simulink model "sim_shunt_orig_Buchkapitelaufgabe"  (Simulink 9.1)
settings: Solver=ode23s  StartTime=0.0  StopTime=4000  RelTol=1e-8  EnableMultiTasking=on
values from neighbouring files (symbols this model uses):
  Bauchdruck = 0    [InitVentil_Buchkapitel.m]
  HydrHoehe = sin(Liegewinkel)*l_Schlauch*73.55    [InitVentil_Buchkapitel.m]
  ICP_n = 0.9330    (= 0.933)    [InitVentil_Buchkapitel.m]
  ICP_shift = 9*sin(Liegewinkel*2 + pi/2)+5 - 14    [InitVentil_Buchkapitel.m]
  R_hyd = 128*eta_Liquor*l_Schlauch/(pi*d_Schlauch^4)*Umrechnungsfaktor    (= 68180382716.6)    [InitVentil_Buchkapitel.m]
  ventil_oeffn = 7    [InitVentil_Buchkapitel.m]
undefined symbols (not defined in the file or in its folder): ABP_n, alph, alphco2, G_vor, h_01, h_02, h_0_ven, ini1_reg, ini2_reg, K_e1, K_e2, K_e_ven, K_G1, K_G2, K_G_ven, k_prod, k_res, K_v1, K_v2, K_v_ven, n_m1, n_m2, O2_verb, p1_n, Pco2_AB, PCO2_soll, Po2_ab, PO2_blut, PO2_soll, r1_100, r2_100, r2_n, r_01, r_02, r_0_ven, r_m1, r_m2, r_t1, r_t2, rv_100, sigma_01, sigma_02, sigma_0_ven, sigma_0_visk_1, sigma_0_visk_2, sigma_koll1, sigma_koll2, sigma_koll_ven, sigma_m01, sigma_m02, V, V1_n, V2_n, V_ven_0, VBPss_n
libraries: neural x36, simulink_extras x3, simulink x1
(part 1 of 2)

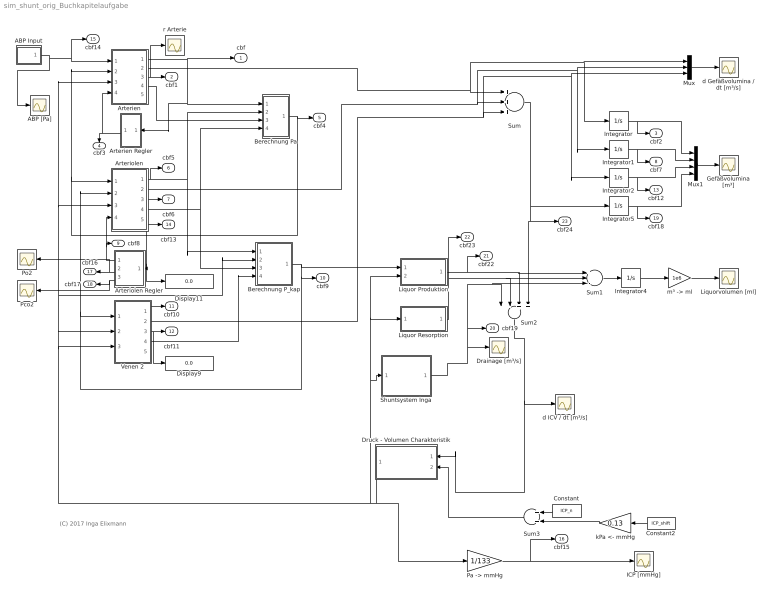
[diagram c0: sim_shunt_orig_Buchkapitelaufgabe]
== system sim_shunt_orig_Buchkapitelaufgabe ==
  note: (C) 2017 Inga Elixmann
  ABP Input : Subsystem
  ABP [Pa] : Scope
  Arterien : Subsystem
  Arterien Regler : Subsystem
  Arteriolen : Subsystem
  Arteriolen Regler : Subsystem
  Berechnung P_kap : Subsystem
  Berechnung Pa : Subsystem
  Constant : Constant  Value=ICP_n
  Constant2 : Constant  Value=ICP_shift
  Display11 : Display
  Display9 : Display
  Drainage [m³/s] : Scope
  Druck - Volumen Charakteristik : Subsystem
  Gefäßvolumina [m³] : Scope
  ICP [mmHg] : Scope
  Integrator : Integrator  InitialCondition=V1_n*1e-6
  Integrator1 : Integrator  InitialCondition=V2_n*1e-6
  Integrator2 : Integrator  InitialCondition=V_ven_0*1e-6
  Integrator4 : Integrator  InitialCondition=150*1e-6
  Integrator5 : Integrator  InitialCondition=(V_ven_0+V2_n+V1_n)*1e-6
  Liquor Produktion : Subsystem
  Liquor Resorption : Subsystem
  Liquorvolumen [ml] : Scope
  Mux : Mux  Inputs=3
  Mux1 : Mux
  "Pa -> mmHg" : Gain  Gain=1/133
  Pco2 : Scope
  Po2 : Scope
  Shuntsystem Inga : Subsystem
  Sum : Sum  Inputs=+++
  Sum1 : Sum  Inputs=+--
  Sum2 : Sum  Inputs=--++
  Sum3 : Sum
  Venen 2 : Subsystem
  d Gefäßvolumina / dt [m³/s] : Scope
  d ICV / dt [m³/s] : Scope
  kPa <- mmHg : Gain  Gain=0.13
  "m³ -> ml" : Gain  Gain=1e6
  r Arterie : Scope
  cbf : Outport
  cbf1 : Outport  Port=2
  cbf2 : Outport  Port=3
  cbf3 : Outport  Port=4
  cbf4 : Outport  Port=5
  cbf5 : Outport  Port=6
  cbf6 : Outport  Port=7
  cbf7 : Outport  Port=8
  cbf8 : Outport  Port=9
  cbf9 : Outport  Port=10
  cbf10 : Outport  Port=11
  cbf11 : Outport  Port=12
  cbf12 : Outport  Port=13
  cbf13 : Outport  Port=14
  cbf14 : Outport  Port=15
  cbf15 : Outport  Port=16
  cbf16 : Outport  Port=17
  cbf17 : Outport  Port=18
  cbf18 : Outport  Port=19
  cbf19 : Outport  Port=20
  cbf22 : Outport  Port=21
  cbf23 : Outport  Port=22
  cbf24 : Outport  Port=23
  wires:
  Arterien/4(G1) -> Berechnung Pa/3(G1)
  Arteriolen/4(G2) -> Berechnung Pa/4(G2), Berechnung P_kap/3(G2)
  Arterien/3(r1) -> cbf1/1, r Arterie/1
  Arterien Regler/1(A1) -> Arterien/4(A), cbf3/1
  Berechnung Pa/1(Pa) -> cbf4/1, Arterien/2(P2), Arteriolen/1(P1)
  Arteriolen/1(PI2) -> Berechnung Pa/2(PI2), Berechnung P_kap/1(PI2), cbf5/1
  Arteriolen/3(r2) -> cbf6/1
  Venen 2/1(PI_ven) -> cbf10/1
  ABP Input/1(ABP) -> Arterien/1(P1), cbf14/1, ABP [Pa]/1
  Venen 2/3(r_ven) -> cbf11/1, Display9/1
  Integrator/1 -> cbf2/1, Mux1/1
  Arterien/2(dV1) -> Sum/1, Mux/1, Integrator/1
  Integrator1/1 -> cbf7/1, Mux1/2
  Arteriolen/2(dV2) -> Sum/2, Mux/2, Integrator1/1
  Integrator2/1 -> Mux1/3, cbf12/1
  Venen 2/4(G_ven) -> Berechnung P_kap/4(G_pv)
  Berechnung P_kap/1(P_kap) -> Liquor Produktion/1(P_kap), Venen 2/1(P1), Arteriolen/2(P2), cbf9/1
  Venen 2/2(dV_ven) -> Sum/3, Mux/3, Integrator2/1
  Arteriolen/5(cbf2) -> cbf13/1, Display11/1, Arteriolen Regler/1(CBF)
  Arteriolen Regler/1(A2) -> Arteriolen/4(A), cbf8/1
  Arteriolen Regler/2(Po2) -> cbf16/1, Po2/1
  Arteriolen Regler/3(Pco2) -> cbf17/1, Pco2/1
  Arterien/1(PI1) -> cbf/1, Berechnung Pa/1(PI1), Arterien Regler/1(Pa)
  Druck - Volumen Charakteristik/1(ICP) -> "Pa -> mmHg"/1, Venen 2/2(P2), Arterien/3(ICP), Arteriolen/3(ICP), Berechnung P_kap/2(ICP), Venen 2/3(ICP), Shuntsystem Inga/1(ICP), Liquor Resorption/1(ICP), Liquor Produktion/2(ICP)
  Liquor Produktion/1(dV_prod) -> Sum1/1, Sum2/3, cbf22/1
  Liquor Resorption/1(dV_res) -> Sum1/2, Sum2/2, cbf23/1
  Sum2/1 -> Druck - Volumen Charakteristik/1(dV/dt), d ICV / dt [m³/s]/1
  Sum/1 -> Integrator5/1, Sum2/4, cbf24/1
  Mux/1 -> d Gefäßvolumina / dt [m³/s]/1
  "Pa -> mmHg"/1 -> ICP [mmHg]/1, cbf15/1
  Mux1/1 -> Gefäßvolumina [m³]/1
  Sum1/1 -> Integrator4/1
  Integrator4/1 -> "m³ -> ml"/1
  "m³ -> ml"/1 -> Liquorvolumen [ml]/1
  Integrator5/1 -> cbf18/1, Mux1/4
  Constant/1 -> Sum3/1
  Sum3/1 -> Druck - Volumen Charakteristik/2(ICP_start)
  Constant2/1 -> kPa <- mmHg/1
  kPa <- mmHg/1 -> Sum3/2
  Shuntsystem Inga/1(dV_shunt) -> Drainage [m³/s]/1, Sum1/3, Sum2/1, cbf19/1

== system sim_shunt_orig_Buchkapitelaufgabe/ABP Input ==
  note: Vereinfachte Annahme: konstanter ABP
  ABP Generator : Subsystem
  ABP [kPa] : Display
  Constant : Constant  Value=ABP_n
  Constant1 : Constant
  From Workspace : FromWorkspace  VariableName=[T,U]  SampleTime=0  Interpolate=off  OutputAfterFinalValue=Holding final value
  Manual Switch : ManualSwitch  CurrentSetting=0
  Manual Switch1 : ManualSwitch
  Manual Switch2 : ManualSwitch
  Product : Product
  Slider Gain : simulink/Math Operations/Slider Gain  gain=1  low=0  high=2
  Step : Step  Time=20  Before=1  After=1.3  SampleTime=0
  "kPa -> Pa" : Gain  Gain=1000
  ABP : Outport
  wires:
  Constant/1 -> Slider Gain/1
  Manual Switch/1 -> Product/2
  Slider Gain/1 -> Product/1
  Step/1 -> Manual Switch/1
  Manual Switch1/1 -> Manual Switch/2
  From Workspace/1 -> Manual Switch1/2
  Constant1/1 -> Manual Switch1/1
  Product/1 -> Manual Switch2/1
  ABP Generator/1(ABP) -> Manual Switch2/2
  Manual Switch2/1 -> ABP [kPa]/1, "kPa -> Pa"/1
  "kPa -> Pa"/1 -> ABP/1

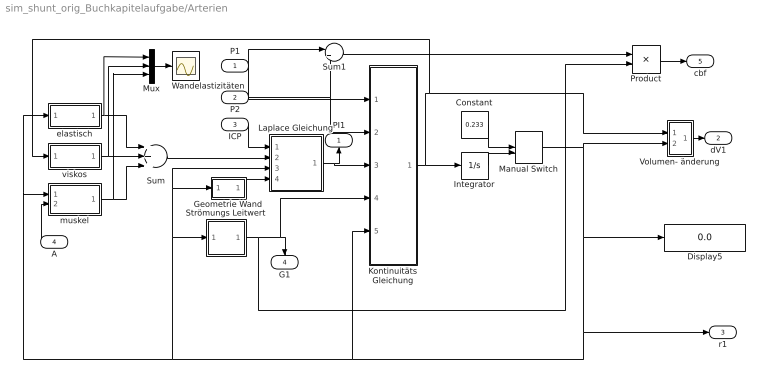
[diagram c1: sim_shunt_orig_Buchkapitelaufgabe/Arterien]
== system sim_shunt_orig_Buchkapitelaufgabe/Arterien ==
  P1 : Inport
  P2 : Inport  Port=2
  ICP : Inport  Port=3
  A : Inport  Port=4
  Constant : Constant  Value=0.233
  Display5 : Display
  Geometrie Wand : Subsystem
  Integrator : Integrator  InitialCondition=r1_100*0.01
  Kontinuitäts Gleichung : Subsystem
  Laplace Gleichung : Subsystem
  Manual Switch : ManualSwitch  CurrentSetting=0
  Mux : Mux  Inputs=3
  Product : Product
  Strömungs Leitwert : Subsystem
  Sum : Sum  Inputs=+++
  Sum1 : Sum  Inputs=|+-
  Volumen- änderung : Subsystem
  Wandelastizitäten : Scope
  elastisch : Subsystem
  muskel : Subsystem
  viskos : Subsystem
  PI1 : Outport
  dV1 : Outport  Port=2
  r1 : Outport  Port=3
  G1 : Outport  Port=4
  cbf : Outport  Port=5
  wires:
  ICP/1 -> Laplace Gleichung/1(ICP)
  Laplace Gleichung/1(PI) -> Kontinuitäts Gleichung/3(PI), PI1/1
  Geometrie Wand/1(h) -> Laplace Gleichung/4(h)
  Constant/1 -> Manual Switch/1
  Integrator/1 -> Manual Switch/2
  Volumen- änderung/1(dV) -> dV1/1
  Manual Switch/1 -> Volumen- änderung/2(r), Strömungs Leitwert/1(r), Geometrie Wand/1(r), Laplace Gleichung/3(r), muskel/1(r), elastisch/1(r), Kontinuitäts Gleichung/5(r), r1/1, Display5/1
  Kontinuitäts Gleichung/1(dr) -> Integrator/1, Volumen- änderung/1(dr), viskos/1(dr)
  A/1 -> muskel/2(A)
  Sum/1 -> Laplace Gleichung/2(Sigma)
  Product/1 -> cbf/1
  P1/1 -> Kontinuitäts Gleichung/1(P1), Sum1/1
  P2/1 -> Kontinuitäts Gleichung/2(P2), Sum1/2
  Sum1/1 -> Product/1
  Strömungs Leitwert/1(G) -> G1/1, Kontinuitäts Gleichung/4(G), Product/2
  elastisch/1(sigma_e) -> Sum/1, Mux/1
  viskos/1(sigma_v) -> Sum/2, Mux/2
  muskel/1(sigma_m) -> Sum/3, Mux/3
  Mux/1 -> Wandelastizitäten/1

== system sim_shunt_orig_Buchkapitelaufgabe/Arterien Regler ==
  Pa : Inport
  CBF Norm : Constant  Value=p1_n
  Display4 : Display
  Gain : Gain  Gain=10
  Gain1 : Gain  Gain=0
  Gain2 : Gain  Gain=1/p1_n
  Integrator1 : Integrator  InitialCondition=ini1_reg  LimitOutput=on  UpperSaturationLimit=100  LowerSaturationLimit=-100
  Mux : Mux  Inputs=3
  "Pa -> kPa" : Gain  Gain=0.001
  Scope : Scope
  Sum1 : Sum  Inputs=|+-
  Sum2 : Sum  Inputs=|++
  Transfer Fcn (with initial outputs) : simulink_extras/Additional Linear/Transfer Fcn (with initial outputs)  N=[1]  D=[2 1]  Y0=A1_100  U0=A1_100
  Transfer Fcn (with initial outputs)1 : simulink_extras/Additional Linear/Transfer Fcn (with initial outputs)  N=[1]  D=[2 1]  Y0=A1_100  U0=A1_100
  logsig2 : neural/Transfer Functions/logsig
  A1 : Outport
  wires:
  Gain/1 -> Sum2/2
  logsig2/1 -> Transfer Fcn (with initial outputs)/1
  Gain1/1 -> Integrator1/1
  Integrator1/1 -> Sum2/1
  Sum2/1 -> logsig2/1, Display4/1
  Transfer Fcn (with initial outputs)1/1 -> A1/1
  Transfer Fcn (with initial outputs)/1 -> Transfer Fcn (with initial outputs)1/1
  Pa/1 -> "Pa -> kPa"/1
  CBF Norm/1 -> Sum1/2, Mux/2
  Sum1/1 -> Gain2/1
  Gain2/1 -> Gain/1, Gain1/1, Mux/3
  Mux/1 -> Scope/1
  "Pa -> kPa"/1 -> Sum1/1, Mux/1

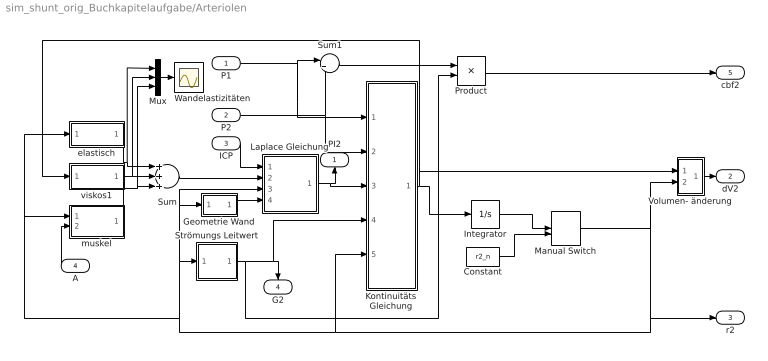
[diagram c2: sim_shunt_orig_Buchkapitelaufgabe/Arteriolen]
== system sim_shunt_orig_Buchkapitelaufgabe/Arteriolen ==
  P1 : Inport
  P2 : Inport  Port=2
  ICP : Inport  Port=3
  A : Inport  Port=4
  Constant : Constant  Value=r2_n
  Geometrie Wand : Subsystem
  Integrator : Integrator  InitialCondition=r2_100*0.01
  Kontinuitäts Gleichung : Subsystem
  Laplace Gleichung : Subsystem
  Manual Switch : ManualSwitch
  Mux : Mux  Inputs=3
  Product : Product
  Strömungs Leitwert : Subsystem
  Sum : Sum  Inputs=+++
  Sum1 : Sum  Inputs=|+-
  Volumen- änderung : Subsystem
  Wandelastizitäten : Scope
  elastisch : Subsystem
  muskel : Subsystem
  viskos1 : Subsystem
  PI2 : Outport
  dV2 : Outport  Port=2
  r2 : Outport  Port=3
  G2 : Outport  Port=4
  cbf2 : Outport  Port=5
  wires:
  Kontinuitäts Gleichung/1(dr) -> Integrator/1, Volumen- änderung/1(dr), viskos1/1(dr)
  Laplace Gleichung/1(PI) -> PI2/1, Kontinuitäts Gleichung/3(PI)
  A/1 -> muskel/2(A)
  ICP/1 -> Laplace Gleichung/1(ICP)
  Geometrie Wand/1(h) -> Laplace Gleichung/4(h)
  Volumen- änderung/1(dV) -> dV2/1
  Manual Switch/1 -> r2/1, muskel/1(r), elastisch/1(r), Laplace Gleichung/3(r), Geometrie Wand/1(r), Strömungs Leitwert/1(r), Kontinuitäts Gleichung/5(r), Volumen- änderung/2(r)
  Integrator/1 -> Manual Switch/1
  Constant/1 -> Manual Switch/2
  elastisch/1(sigma_e) -> Sum/1, Mux/1
  viskos1/1(sigma_v) -> Sum/2, Mux/2
  Sum/1 -> Laplace Gleichung/2(Sigma)
  P2/1 -> Kontinuitäts Gleichung/2(P2), Sum1/2
  P1/1 -> Kontinuitäts Gleichung/1(P1), Sum1/1
  Sum1/1 -> Product/1
  Strömungs Leitwert/1(G) -> G2/1, Kontinuitäts Gleichung/4(G), Product/2
  Product/1 -> cbf2/1
  muskel/1(sigma_m) -> Sum/3, Mux/3
  Mux/1 -> Wandelastizitäten/1

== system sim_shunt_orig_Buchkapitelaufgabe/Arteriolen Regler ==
  CBF : Inport
  CO2 Modell : Subsystem
  Mux : Mux  Inputs=3
  O2 Modell : Subsystem
  Partialdrücke u. CBF [mmHg] bzw. [ml/s] : Scope
  "m³/s -> cm³/s" : Gain  Gain=1e6
  regler : Subsystem
  A2 : Outport
  Po2 : Outport  Port=2
  Pco2 : Outport  Port=3
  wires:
  regler/1(Out1) -> A2/1
  CBF/1 -> "m³/s -> cm³/s"/1
  O2 Modell/1(PO2) -> regler/1(In1), Po2/1, CO2 Modell/2(PO2), Mux/2
  CO2 Modell/1(PCO2) -> Pco2/1, regler/2(In2), Mux/3
  "m³/s -> cm³/s"/1 -> O2 Modell/1(CBF), CO2 Modell/1(CBF), Mux/1
  Mux/1 -> Partialdrücke u. CBF [mmHg] bzw. [ml/s]/1

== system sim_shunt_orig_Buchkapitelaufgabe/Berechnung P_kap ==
  PI2 : Inport
  ICP : Inport  Port=2
  G2 : Inport  Port=3
  G_pv : Inport  Port=4
  Constant Pcap : Constant  Value=2
  Mux : Mux  Inputs=2
  Pa Berechnung : Fcn  Expr=u(2)/(u(1)+u(2))
  Product : Product
  Product1 : Product
  Sum : Sum  Inputs=|+-
  Sum3 : Sum  Inputs=|+-
  P_kap : Outport
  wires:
  Sum3/1 -> P_kap/1
  PI2/1 -> Sum3/1, Sum/1
  Product/1 -> Sum3/2
  G_pv/1 -> Mux/2
  ICP/1 -> Sum/2
  Sum/1 -> Product/1
  Pa Berechnung/1 -> Product/2
  Mux/1 -> Pa Berechnung/1
  Product1/1 -> Mux/1
  G2/1 -> Product1/1
  Constant Pcap/1 -> Product1/2

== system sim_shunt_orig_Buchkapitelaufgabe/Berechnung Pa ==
  PI1 : Inport
  PI2 : Inport  Port=2
  G1 : Inport  Port=3
  G2 : Inport  Port=4
  Mux : Mux  Inputs=2
  Pa Berechnung : Fcn  Expr=u(2)/(u(1)+u(2))
  Product : Product
  Sum : Sum  Inputs=|+-
  Sum3 : Sum  Inputs=|+-
  Pa : Outport
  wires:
  Mux/1 -> Pa Berechnung/1
  Pa Berechnung/1 -> Product/2
  Sum/1 -> Product/1
  PI2/1 -> Sum/2
  G1/1 -> Mux/1
  G2/1 -> Mux/2
  Product/1 -> Sum3/2
  PI1/1 -> Sum/1, Sum3/1
  Sum3/1 -> Pa/1

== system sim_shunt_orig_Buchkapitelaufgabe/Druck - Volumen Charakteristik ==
  dV/dt : Inport
  ICP_start : Inport  Port=2
  Integrator3 : Integrator  InitialConditionSource=external  InitialCondition=ICP_n
  Pa <- kPa : Gain  Gain=1000
  Product : Product
  k_elast gesund: 0,11 1/ml pathologisch: 0,26 1/ml : Gain  Gain=0.26
  "m³ -> cm³ = ml" : Gain  Gain=1e6
  ICP : Outport
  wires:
  k_elast gesund: 0,11 1/ml pathologisch: 0,26 1/ml/1 -> Product/1
  Product/1 -> Integrator3/1
  "m³ -> cm³ = ml"/1 -> k_elast gesund: 0,11 1/ml pathologisch: 0,26 1/ml/1
  Integrator3/1 -> Pa <- kPa/1, Product/2
  dV/dt/1 -> "m³ -> cm³ = ml"/1
  Pa <- kPa/1 -> ICP/1
  ICP_start/1 -> Integrator3/2

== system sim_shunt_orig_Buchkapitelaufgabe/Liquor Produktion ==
  P_kap : Inport
  ICP : Inport  Port=2
  Gain1 : Gain  Gain=k_prod
  Sum1 : Sum  Inputs=|+-
  "µl -> m³" : Gain  Gain=1e-9
  dV_prod : Outport
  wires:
  Gain1/1 -> "µl -> m³"/1
  P_kap/1 -> Sum1/1
  Sum1/1 -> Gain1/1
  ICP/1 -> Sum1/2
  "µl -> m³"/1 -> dV_prod/1

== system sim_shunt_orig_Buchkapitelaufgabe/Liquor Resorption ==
  ICP : Inport
  Constant2 : Constant  Value=VBPss_n
  Constant3 : Constant  Value=0
  Gain1 k_res - gesund k_res/3 - BWellen k_res/12 - AWellen : Gain  Gain=k_res/3
  Sum1 : Sum  Inputs=|+-
  Switch : Switch
  kPa->Pa : Gain  Gain=1000
  "µl -> m³" : Gain  Gain=1e-9
  dV_res : Outport
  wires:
  Constant2/1 -> kPa->Pa/1
  Sum1/1 -> Gain1 k_res - gesund k_res/3 - BWellen k_res/12 - AWellen/1
  ICP/1 -> Sum1/1
  Switch/1 -> dV_res/1
  Gain1 k_res - gesund k_res/3 - BWellen k_res/12 - AWellen/1 -> "µl -> m³"/1
  Constant3/1 -> Switch/3
  kPa->Pa/1 -> Sum1/2
  "µl -> m³"/1 -> Switch/1, Switch/2

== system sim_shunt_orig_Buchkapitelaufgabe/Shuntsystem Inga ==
  ICP : Inport
  Constant2 : Constant  Value=ventil_oeffn
  Constant4 : Constant  Value=Bauchdruck
  Constant5 : Constant  Value=HydrHoehe
  "Pa -> mmHg" : Gain  Gain=1/133
  Sum1 : Sum  Inputs=-++
  Sum2 : Sum  Inputs=|+-
  Sum8 : Sum  Inputs=|++
  ml/mmHg : Gain  Gain=R_hyd
  "ml/s -> m³/s" : Gain  Gain=1/1000
  dV_shunt : Outport
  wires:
  ICP/1 -> "Pa -> mmHg"/1
  ml/mmHg/1 -> "ml/s -> m³/s"/1
  Sum1/1 -> ml/mmHg/1
  "Pa -> mmHg"/1 -> Sum2/1
  Constant4/1 -> Sum2/2
  Constant2/1 -> Sum1/1
  Sum2/1 -> Sum8/1
  Sum8/1 -> Sum1/2
  Constant5/1 -> Sum8/2
  "ml/s -> m³/s"/1 -> dV_shunt/1

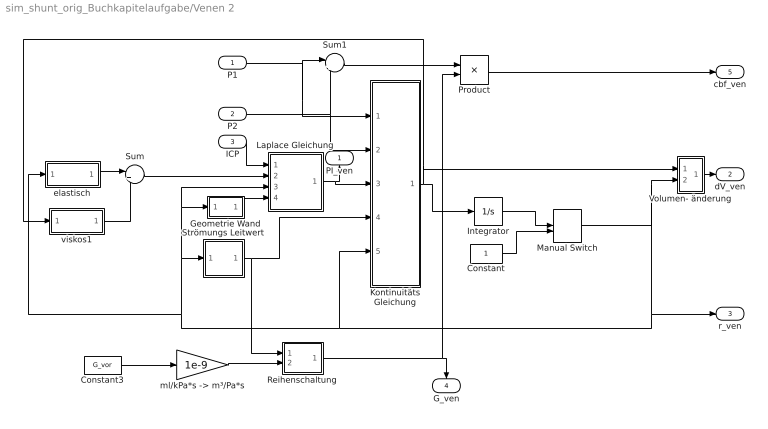
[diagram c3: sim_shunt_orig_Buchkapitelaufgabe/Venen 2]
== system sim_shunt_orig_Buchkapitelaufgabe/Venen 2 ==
  P1 : Inport
  P2 : Inport  Port=2
  ICP : Inport  Port=3
  Constant : Constant
  Constant3 : Constant  Value=G_vor
  Geometrie Wand : Subsystem
  Integrator : Integrator  InitialCondition=rv_100*0.01  LimitOutput=on  UpperSaturationLimit=1000  LowerSaturationLimit=-1000
  Kontinuitäts Gleichung : Subsystem
  Laplace Gleichung : Subsystem
  Manual Switch : ManualSwitch
  Product : Product
  Reihenschaltung : Subsystem
  Strömungs Leitwert : Subsystem
  Sum : Sum  Inputs=|++
  Sum1 : Sum  Inputs=|+-
  Volumen- änderung : Subsystem
  elastisch : Subsystem
  "ml/kPa*s -> m³/Pa*s" : Gain  Gain=1e-9
  viskos1 : Subsystem
  PI_ven : Outport
  dV_ven : Outport  Port=2
  r_ven : Outport  Port=3
  G_ven : Outport  Port=4
  cbf_ven : Outport  Port=5
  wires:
  Constant3/1 -> "ml/kPa*s -> m³/Pa*s"/1
  Strömungs Leitwert/1(G) -> Reihenschaltung/1(G1), Kontinuitäts Gleichung/4(G)
  Kontinuitäts Gleichung/1(dr) -> Integrator/1, Volumen- änderung/1(dr), viskos1/1(dr)
  Laplace Gleichung/1(PI) -> PI_ven/1, Kontinuitäts Gleichung/3(PI)
  ICP/1 -> Laplace Gleichung/1(ICP)
  Geometrie Wand/1(h) -> Laplace Gleichung/4(h)
  Volumen- änderung/1(dV) -> dV_ven/1
  Manual Switch/1 -> Volumen- änderung/2(r), r_ven/1, elastisch/1(r), Laplace Gleichung/3(r), Geometrie Wand/1(r), Strömungs Leitwert/1(r), Kontinuitäts Gleichung/5(r)
  Integrator/1 -> Manual Switch/1
  Constant/1 -> Manual Switch/2
  P2/1 -> Kontinuitäts Gleichung/2(P2), Sum1/2
  P1/1 -> Kontinuitäts Gleichung/1(P1), Sum1/1
  Sum1/1 -> Product/1
  Product/1 -> cbf_ven/1
  Reihenschaltung/1(G_ges) -> Product/2, G_ven/1
  elastisch/1(sigma_e) -> Sum/1
  Sum/1 -> Laplace Gleichung/2(Sigma)
  viskos1/1(sigma_v) -> Sum/2
  "ml/kPa*s -> m³/Pa*s"/1 -> Reihenschaltung/2(G2)

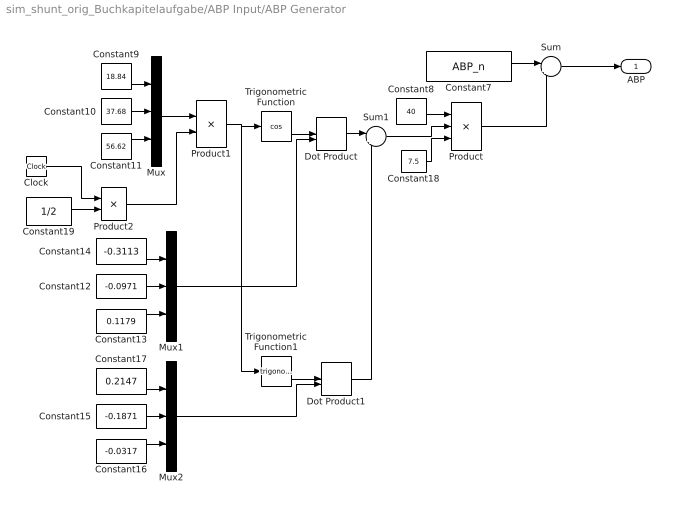
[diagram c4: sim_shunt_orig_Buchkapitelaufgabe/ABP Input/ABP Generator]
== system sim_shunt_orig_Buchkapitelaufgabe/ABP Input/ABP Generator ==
  Clock : Clock
  Constant10 : Constant  Value=37.68
  Constant11 : Constant  Value=56.62
  Constant12 : Constant  Value=-0.0971
  Constant13 : Constant  Value=0.1179
  Constant14 : Constant  Value=-0.3113
  Constant15 : Constant  Value=-0.1871
  Constant16 : Constant  Value=-0.0317
  Constant17 : Constant  Value=0.2147
  Constant18 : Constant  Value=7.5
  Constant19 : Constant  Value=1/2
  Constant7 : Constant  Value=ABP_n
  Constant8 : Constant  Value=40
  Constant9 : Constant  Value=18.84
  Dot Product : DotProduct
  Dot Product1 : DotProduct
  Mux : Mux  Inputs=3
  Mux1 : Mux  Inputs=3
  Mux2 : Mux  Inputs=3
  Product : Product  Inputs=**/
  Product1 : Product
  Product2 : Product
  Sum : Sum  Inputs=|++
  Sum1 : Sum  Inputs=|++
  Trigonometric Function : Trigonometry  Operator=cos
  Trigonometric Function1 : Trigonometry
  ABP : Outport
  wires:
  Clock/1 -> Product2/1
  Constant15/1 -> Mux2/2
  Constant16/1 -> Mux2/3
  Constant14/1 -> Mux1/1
  Constant19/1 -> Product2/2
  Product2/1 -> Product1/2
  Sum1/1 -> Product/2
  Constant8/1 -> Product/1
  Dot Product1/1 -> Sum1/2
  Dot Product/1 -> Sum1/1
  Mux1/1 -> Dot Product/2
  Constant13/1 -> Mux1/3
  Constant12/1 -> Mux1/2
  Mux2/1 -> Dot Product1/2
  Constant17/1 -> Mux2/1
  Product1/1 -> Trigonometric Function1/1, Trigonometric Function/1
  Trigonometric Function1/1 -> Dot Product1/1
  Trigonometric Function/1 -> Dot Product/1
  Mux/1 -> Product1/1
  Constant11/1 -> Mux/3
  Constant10/1 -> Mux/2
  Constant9/1 -> Mux/1
  Constant18/1 -> Product/3
  Sum/1 -> ABP/1
  Product/1 -> Sum/2
  Constant7/1 -> Sum/1

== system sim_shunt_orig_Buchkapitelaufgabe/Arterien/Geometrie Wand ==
  r : Inport
  " " : Math  Operator=square
  "  " : Product  Inputs=***
  Faktor : Constant  Value=2
  Summe : Sum  Inputs=+++
  Wurzel : Math  Operator=sqrt
  cm --> m : Gain  Gain=0.01
  "cm -> m" : Gain  Gain=0.01
  "h_1 " : Sum  Inputs=+-
  ho_1 : Constant  Value=h_01
  r ^ 2 : Math  Operator=square
  ro_1 : Constant  Value=r_01
  h : Outport
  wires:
  r/1 -> "h_1 "/2, r ^ 2/1
  Summe/1 -> Wurzel/1
  Wurzel/1 -> "h_1 "/1
  r ^ 2/1 -> Summe/3
  " "/1 -> Summe/2
  ho_1/1 -> cm --> m/1
  ro_1/1 -> "cm -> m"/1
  Faktor/1 -> "  "/1
  "  "/1 -> Summe/1
  "h_1 "/1 -> h/1
  "cm -> m"/1 -> "  "/2
  cm --> m/1 -> " "/1, "  "/3

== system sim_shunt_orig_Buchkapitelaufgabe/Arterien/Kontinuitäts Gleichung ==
  P1 : Inport
  P2 : Inport  Port=2
  PI : Inport  Port=3
  G : Inport  Port=4
  r : Inport  Port=5
  2 Korrekturfaktor : Gain
  Constant2 : Constant  Value=K_v1
  Product1 : Product
  Product2 : Product  Inputs=*//
  Sum : Sum  Inputs=|+-
  Sum1 : Sum  Inputs=|+-
  Sum2 : Sum  Inputs=|+-
  "cm -> m" : Gain  Gain=0.01
  dr : Outport
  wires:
  P1/1 -> Sum/1
  P2/1 -> Sum1/2
  Sum/1 -> Sum2/1
  Sum1/1 -> Sum2/2
  Sum2/1 -> Product1/1
  Product2/1 -> dr/1
  r/1 -> Product2/3
  Constant2/1 -> "cm -> m"/1
  Product1/1 -> Product2/1
  G/1 -> Product1/2
  PI/1 -> Sum/2, Sum1/1
  "cm -> m"/1 -> 2 Korrekturfaktor/1
  2 Korrekturfaktor/1 -> Product2/2

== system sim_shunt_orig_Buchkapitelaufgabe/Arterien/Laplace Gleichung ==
  ICP : Inport
  Sigma : Inport  Port=2
  r : Inport  Port=3
  h : Inport  Port=4
  " " : Product  Inputs=**
  "  P_1" : Product  Inputs=*/
  " 1" : Product  Inputs=**
  Summe : Sum
  r +h : Sum
  PI : Outport
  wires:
  "  P_1"/1 -> PI/1
  Summe/1 -> "  P_1"/1
  r +h/1 -> " "/2
  ICP/1 -> " "/1
  " "/1 -> Summe/2
  r/1 -> "  P_1"/2, r +h/1
  Sigma/1 -> " 1"/1
  h/1 -> r +h/2, " 1"/2
  " 1"/1 -> Summe/1

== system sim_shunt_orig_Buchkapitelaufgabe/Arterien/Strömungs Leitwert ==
  r : Inport
  "1/kPa*cm*s -> 1/Pa*m*s" : Gain  Gain=0.1
  Leitwert Konstante : Constant  Value=K_G1
  Potenz : Constant  Value=4
  Product : Product
  r ^ 4 : Math  Operator=pow
  G : Outport
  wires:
  Potenz/1 -> r ^ 4/2
  r ^ 4/1 -> Product/1
  Leitwert Konstante/1 -> "1/kPa*cm*s -> 1/Pa*m*s"/1
  r/1 -> r ^ 4/1
  Product/1 -> G/1
  "1/kPa*cm*s -> 1/Pa*m*s"/1 -> Product/2

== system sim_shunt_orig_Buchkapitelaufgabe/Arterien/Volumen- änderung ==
  dr : Inport
  r : Inport  Port=2
  2 Korrekturfaktor : Gain
  Faktor : Constant  Value=2
  Kv_1 : Constant  Value=K_v1
  "cm -> m" : Gain  Gain=0.01
  "dV_1 " : Product  Inputs=4
  dV : Outport
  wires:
  r/1 -> "dV_1 "/4
  dr/1 -> "dV_1 "/3
  Kv_1/1 -> "cm -> m"/1
  Faktor/1 -> "dV_1 "/1
  "dV_1 "/1 -> dV/1
  "cm -> m"/1 -> 2 Korrekturfaktor/1
  2 Korrekturfaktor/1 -> "dV_1 "/2

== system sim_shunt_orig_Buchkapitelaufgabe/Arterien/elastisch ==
  r : Inport
  (r-r0) / r0 : Product  Inputs=**/
  (r-r0) / r1 : Product
  Constant : Constant  Value=r_01
  Constant1 : Constant  Value=sigma_01
  Constant2 : Constant  Value=sigma_koll1
  Constant3 : Constant  Value=K_e1
  Constant4 : Constant
  Sum : Sum  Inputs=|+-
  Sum1 : Sum  Inputs=|+-
  Sum2 : Sum  Inputs=|+-
  "cm -> m" : Gain  Gain=0.01
  dyn*cm^-2 --> Pa : Gain  Gain=0.1
  "dyn*cm^-2 -> Pa" : Gain  Gain=0.1
  r ^ 4 : Math
  sigma_e : Outport
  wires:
  r/1 -> Sum/1
  (r-r0) / r0/1 -> r ^ 4/1
  Constant2/1 -> dyn*cm^-2 --> Pa/1
  Sum1/1 -> sigma_e/1
  Constant/1 -> "cm -> m"/1
  Constant3/1 -> (r-r0) / r0/1
  Sum/1 -> (r-r0) / r0/2
  Constant1/1 -> "dyn*cm^-2 -> Pa"/1
  (r-r0) / r1/1 -> Sum1/1
  r ^ 4/1 -> Sum2/1
  Sum2/1 -> (r-r0) / r1/1
  Constant4/1 -> Sum2/2
  "dyn*cm^-2 -> Pa"/1 -> (r-r0) / r1/2
  dyn*cm^-2 --> Pa/1 -> Sum1/2
  "cm -> m"/1 -> Sum/2, (r-r0) / r0/3

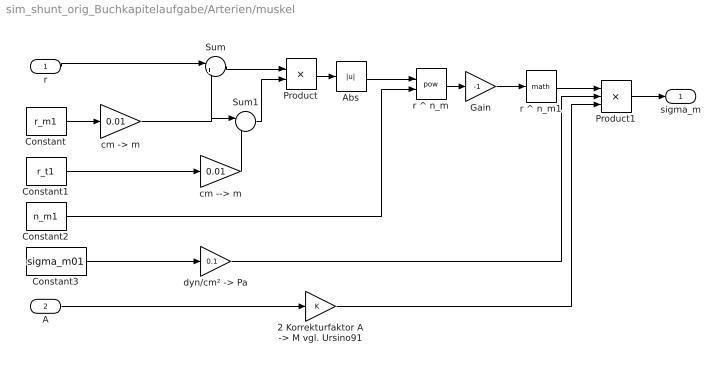
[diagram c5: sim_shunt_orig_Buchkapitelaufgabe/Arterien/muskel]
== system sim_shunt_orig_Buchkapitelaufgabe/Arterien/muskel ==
  r : Inport
  A : Inport  Port=2
  "2 Korrekturfaktor A -> M vgl. Ursino91" : Gain
  Abs : Abs
  Constant : Constant  Value=r_m1
  Constant1 : Constant  Value=r_t1
  Constant2 : Constant  Value=n_m1
  Constant3 : Constant  Value=sigma_m01
  Gain : Gain  Gain=-1
  Product : Product  Inputs=*/
  Product1 : Product  Inputs=3
  Sum : Sum  Inputs=|+-
  Sum1 : Sum  Inputs=|-+
  cm --> m : Gain  Gain=0.01
  "cm -> m" : Gain  Gain=0.01
  "dyn/cm² -> Pa" : Gain  Gain=0.1
  r ^ n_m : Math  Operator=pow
  r ^ n_m1 : Math
  sigma_m : Outport
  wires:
  Sum/1 -> Product/1
  r/1 -> Sum/1
  Constant1/1 -> cm --> m/1
  Sum1/1 -> Product/2
  Product/1 -> Abs/1
  Abs/1 -> r ^ n_m/1
  Constant2/1 -> r ^ n_m/2
  r ^ n_m/1 -> Gain/1
  Gain/1 -> r ^ n_m1/1
  r ^ n_m1/1 -> Product1/1
  Constant3/1 -> "dyn/cm² -> Pa"/1
  A/1 -> "2 Korrekturfaktor A -> M vgl. Ursino91"/1
  Product1/1 -> sigma_m/1
  Constant/1 -> "cm -> m"/1
  "cm -> m"/1 -> Sum/2, Sum1/1
  cm --> m/1 -> Sum1/2
  "2 Korrekturfaktor A -> M vgl. Ursino91"/1 -> Product1/3
  "dyn/cm² -> Pa"/1 -> Product1/2

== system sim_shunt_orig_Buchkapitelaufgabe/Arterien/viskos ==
  dr : Inport
  Constant2 : Constant  Value=sigma_0_visk_1
  Product : Product
  Transfer Fcn : TransferFcn  Denominator=[0.01 1]
  "dyn*s/cm³ -> Pa*s/m" : Gain  Gain=10
  sigma_v : Outport
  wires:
  Product/1 -> sigma_v/1
  dr/1 -> Transfer Fcn/1
  Constant2/1 -> "dyn*s/cm³ -> Pa*s/m"/1
  Transfer Fcn/1 -> Product/1
  "dyn*s/cm³ -> Pa*s/m"/1 -> Product/2

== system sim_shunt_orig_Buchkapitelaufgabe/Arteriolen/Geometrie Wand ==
  r : Inport
  " " : Math  Operator=square
  "  " : Product  Inputs=***
  Faktor : Constant  Value=2
  Summe : Sum  Inputs=+++
  Wurzel : Math  Operator=sqrt
  cm --> m : Gain  Gain=0.01
  "cm -> m" : Gain  Gain=0.01
  "h_1 " : Sum  Inputs=+-
  ho_1 : Constant  Value=h_02
  r ^ 2 : Math  Operator=square
  ro_1 : Constant  Value=r_02
  h : Outport
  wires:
  "h_1 "/1 -> h/1
  "  "/1 -> Summe/1
  Faktor/1 -> "  "/1
  ro_1/1 -> "cm -> m"/1
  ho_1/1 -> cm --> m/1
  " "/1 -> Summe/2
  r ^ 2/1 -> Summe/3
  Wurzel/1 -> "h_1 "/1
  Summe/1 -> Wurzel/1
  r/1 -> r ^ 2/1, "h_1 "/2
  "cm -> m"/1 -> "  "/2
  cm --> m/1 -> "  "/3, " "/1

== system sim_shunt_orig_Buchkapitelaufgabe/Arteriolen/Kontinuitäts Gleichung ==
  P1 : Inport
  P2 : Inport  Port=2
  PI : Inport  Port=3
  G : Inport  Port=4
  r : Inport  Port=5
  0.5 Korrekturfaktor V_aio = 3.5 cm³ : Gain
  Constant2 : Constant  Value=K_v2
  Product1 : Product
  Product2 : Product  Inputs=*//
  Sum : Sum  Inputs=|+-
  Sum1 : Sum  Inputs=|+-
  Sum2 : Sum  Inputs=|+-
  "cm -> m" : Gain  Gain=0.01
  dr : Outport
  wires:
  PI/1 -> Sum1/1, Sum/2
  G/1 -> Product1/2
  Product1/1 -> Product2/1
  Constant2/1 -> "cm -> m"/1
  r/1 -> Product2/3
  Product2/1 -> dr/1
  Sum2/1 -> Product1/1
  Sum1/1 -> Sum2/2
  Sum/1 -> Sum2/1
  P2/1 -> Sum1/2
  P1/1 -> Sum/1
  "cm -> m"/1 -> 0.5 Korrekturfaktor V_aio = 3.5 cm³/1
  0.5 Korrekturfaktor V_aio = 3.5 cm³/1 -> Product2/2

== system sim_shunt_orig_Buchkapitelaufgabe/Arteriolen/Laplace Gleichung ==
  ICP : Inport
  Sigma : Inport  Port=2
  r : Inport  Port=3
  h : Inport  Port=4
  " " : Product  Inputs=**
  "  P_1" : Product  Inputs=*/
  " 1" : Product  Inputs=**
  Summe : Sum
  r +h : Sum
  PI : Outport
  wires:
  h/1 -> " 1"/2, r +h/2
  Sigma/1 -> " 1"/1
  r/1 -> r +h/1, "  P_1"/2
  ICP/1 -> " "/1
  r +h/1 -> " "/2
  "  P_1"/1 -> PI/1
  " 1"/1 -> Summe/1
  Summe/1 -> "  P_1"/1
  " "/1 -> Summe/2

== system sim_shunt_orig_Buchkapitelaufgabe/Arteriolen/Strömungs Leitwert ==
  r : Inport
  1/kPa*cm*s in 1/Pa*m*s : Gain  Gain=0.1
  Leitwert Konstante : Constant  Value=K_G2
  Potenz : Constant  Value=4
  Product : Product
  r ^ 4 : Math  Operator=pow
  G : Outport
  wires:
  Product/1 -> G/1
  r/1 -> r ^ 4/1
  Leitwert Konstante/1 -> 1/kPa*cm*s in 1/Pa*m*s/1
  r ^ 4/1 -> Product/1
  Potenz/1 -> r ^ 4/2
  1/kPa*cm*s in 1/Pa*m*s/1 -> Product/2

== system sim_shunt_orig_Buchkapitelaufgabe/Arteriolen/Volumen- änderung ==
  dr : Inport
  r : Inport  Port=2
  0.5 Korrekturfaktor : Gain
  Faktor : Constant  Value=2
  Kv_1 : Constant  Value=K_v2
  "cm -> m" : Gain  Gain=0.01
  "dV_1 " : Product  Inputs=4
  dV : Outport
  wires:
  "dV_1 "/1 -> dV/1
  Faktor/1 -> "dV_1 "/1
  Kv_1/1 -> "cm -> m"/1
  dr/1 -> "dV_1 "/3
  r/1 -> "dV_1 "/4
  "cm -> m"/1 -> 0.5 Korrekturfaktor/1
  0.5 Korrekturfaktor/1 -> "dV_1 "/2

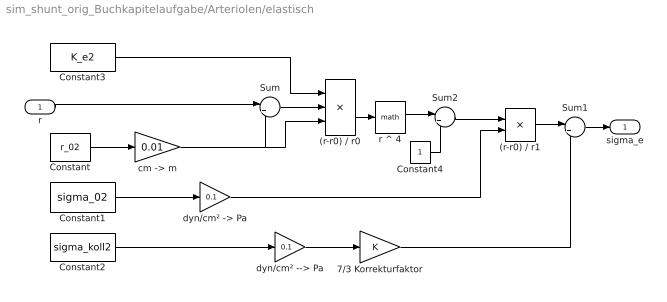
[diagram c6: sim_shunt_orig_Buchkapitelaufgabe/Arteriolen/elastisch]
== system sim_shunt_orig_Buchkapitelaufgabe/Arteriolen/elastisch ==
  r : Inport
  (r-r0) / r0 : Product  Inputs=**/
  (r-r0) / r1 : Product
  7/3 Korrekturfaktor : Gain
  Constant : Constant  Value=r_02
  Constant1 : Constant  Value=sigma_02
  Constant2 : Constant  Value=sigma_koll2
  Constant3 : Constant  Value=K_e2
  Constant4 : Constant
  Sum : Sum  Inputs=|+-
  Sum1 : Sum  Inputs=|+-
  Sum2 : Sum  Inputs=|+-
  "cm -> m" : Gain  Gain=0.01
  dyn/cm² --> Pa : Gain  Gain=0.1
  "dyn/cm² -> Pa" : Gain  Gain=0.1
  r ^ 4 : Math
  sigma_e : Outport
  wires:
  Sum/1 -> (r-r0) / r0/2
  Constant3/1 -> (r-r0) / r0/1
  Constant/1 -> "cm -> m"/1
  (r-r0) / r0/1 -> r ^ 4/1
  r/1 -> Sum/1
  Sum1/1 -> sigma_e/1
  Constant2/1 -> dyn/cm² --> Pa/1
  (r-r0) / r1/1 -> Sum1/1
  Constant1/1 -> "dyn/cm² -> Pa"/1
  r ^ 4/1 -> Sum2/1
  Sum2/1 -> (r-r0) / r1/1
  Constant4/1 -> Sum2/2
  "cm -> m"/1 -> (r-r0) / r0/3, Sum/2
  "dyn/cm² -> Pa"/1 -> (r-r0) / r1/2
  dyn/cm² --> Pa/1 -> 7/3 Korrekturfaktor/1
  7/3 Korrekturfaktor/1 -> Sum1/2

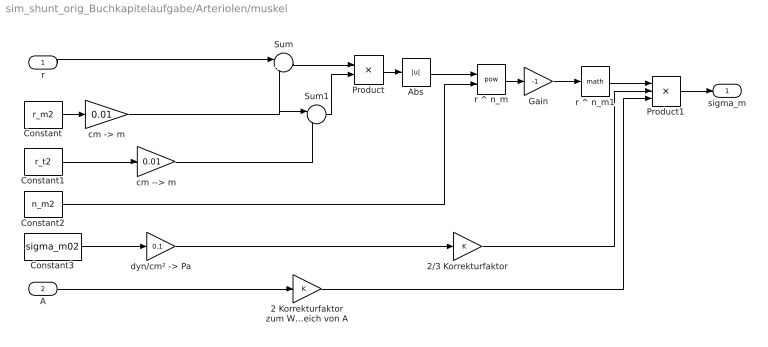
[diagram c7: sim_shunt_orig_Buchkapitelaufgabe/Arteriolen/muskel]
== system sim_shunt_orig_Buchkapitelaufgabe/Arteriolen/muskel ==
  r : Inport
  A : Inport  Port=2
  2 Korrekturfaktor zum Wertebereich von A : Gain
  2/3 Korrekturfaktor : Gain
  Abs : Abs
  Constant : Constant  Value=r_m2
  Constant1 : Constant  Value=r_t2
  Constant2 : Constant  Value=n_m2
  Constant3 : Constant  Value=sigma_m02
  Gain : Gain  Gain=-1
  Product : Product  Inputs=*/
  Product1 : Product  Inputs=3
  Sum : Sum  Inputs=|+-
  Sum1 : Sum  Inputs=|-+
  cm --> m : Gain  Gain=0.01
  "cm -> m" : Gain  Gain=0.01
  "dyn/cm² -> Pa" : Gain  Gain=0.1
  r ^ n_m : Math  Operator=pow
  r ^ n_m1 : Math
  sigma_m : Outport
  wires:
  Product1/1 -> sigma_m/1
  A/1 -> 2 Korrekturfaktor zum Wertebereich von A/1
  Constant3/1 -> "dyn/cm² -> Pa"/1
  r ^ n_m1/1 -> Product1/1
  Gain/1 -> r ^ n_m1/1
  r ^ n_m/1 -> Gain/1
  Constant2/1 -> r ^ n_m/2
  Abs/1 -> r ^ n_m/1
  Product/1 -> Abs/1
  Sum1/1 -> Product/2
  Constant1/1 -> cm --> m/1
  Constant/1 -> "cm -> m"/1
  r/1 -> Sum/1
  Sum/1 -> Product/1
  "cm -> m"/1 -> Sum1/1, Sum/2
  cm --> m/1 -> Sum1/2
  "dyn/cm² -> Pa"/1 -> 2/3 Korrekturfaktor/1
  2/3 Korrekturfaktor/1 -> Product1/2
  2 Korrekturfaktor zum Wertebereich von A/1 -> Product1/3

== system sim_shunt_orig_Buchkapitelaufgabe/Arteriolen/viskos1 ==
  dr : Inport
  Constant2 : Constant  Value=sigma_0_visk_2
  Product : Product
  Transfer Fcn : TransferFcn  Denominator=[0.01 1]
  "dyn*s/cm³ -> Pa*s/m" : Gain  Gain=10
  sigma_v : Outport
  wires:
  Transfer Fcn/1 -> Product/1
  Constant2/1 -> "dyn*s/cm³ -> Pa*s/m"/1
  dr/1 -> Transfer Fcn/1
  Product/1 -> sigma_v/1
  "dyn*s/cm³ -> Pa*s/m"/1 -> Product/2

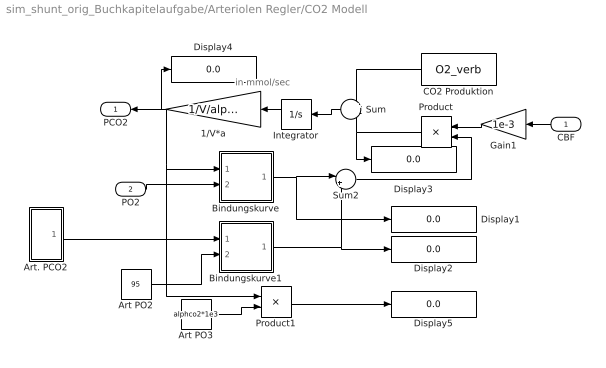
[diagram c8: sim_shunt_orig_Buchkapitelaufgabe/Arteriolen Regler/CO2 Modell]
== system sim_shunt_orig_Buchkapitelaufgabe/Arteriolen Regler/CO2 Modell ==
  note: in mmol/sec
  CBF : Inport
  PO2 : Inport  Port=2
  1/V*a : Gain  Gain=1/V/alphco2
  Art PO2 : Constant  Value=95
  Art PO3 : Constant  Value=alphco2*1e3
  Art. PCO2 : Subsystem
  Bindungskurve : Subsystem
  Bindungskurve1 : Subsystem
  CO2 Produktion : Constant  Value=O2_verb
  Display{1..5} (5 alike) : Display
  Gain1 : Gain  Gain=1e-3
  Integrator : Integrator  InitialCondition=Pco2_AB*V*alphco2  LimitOutput=on  LowerSaturationLimit=0
  Product : Product
  Product1 : Product
  Sum : Sum  Inputs=+-
  Sum2 : Sum  Inputs=|+-
  PCO2 : Outport
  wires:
  Product1/1 -> Display5/1
  Art PO3/1 -> Product1/2
  1/V*a/1 -> Product1/1, Bindungskurve/1(PCO2), Display4/1, PCO2/1
  Product/1 -> Display3/1, Sum/2
  Bindungskurve/1(MCO2) -> Display1/1, Sum2/1
  Bindungskurve1/1(MCO2) -> Display2/1, Sum2/2
  Sum2/1 -> Product/2
  Art PO2/1 -> Bindungskurve1/2(PO2)
  PO2/1 -> Bindungskurve/2(PO2)
  Gain1/1 -> Product/1
  Integrator/1 -> 1/V*a/1
  Sum/1 -> Integrator/1
  CO2 Produktion/1 -> Sum/1
  CBF/1 -> Gain1/1
  Art. PCO2/1(Out1) -> Bindungskurve1/1(PCO2)

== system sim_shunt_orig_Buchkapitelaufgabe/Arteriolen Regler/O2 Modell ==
  note: in mmol/sec
  note: mmol/s
  note: mmol/s
  note: ml/s
  note: mmHg
  note: mol/ml ?
  note: mmHg
  CBF : Inport
  1/(V*a) : Gain  Gain=1/V/alph
  Art PO2 : Constant  Value=PO2_blut
  Gain1 : Gain  Gain=1e-3
  HB Bindung : Subsystem
  HB Bindung1 : Subsystem
  Integrator : Integrator  InitialCondition=Po2_ab*V*alph  LimitOutput=on  LowerSaturationLimit=0
  O2 Verbrauch : Constant  Value=O2_verb
  Product : Product
  Sum : Sum  Inputs=-+
  Sum1 : Sum  Inputs=|-+
  PO2 : Outport
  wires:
  1/(V*a)/1 -> HB Bindung1/1(PO2), PO2/1
  O2 Verbrauch/1 -> Sum/1
  CBF/1 -> Gain1/1
  Sum1/1 -> Product/2
  Integrator/1 -> 1/(V*a)/1
  Gain1/1 -> Product/1
  HB Bindung/1(MO2) -> Sum1/2
  HB Bindung1/1(MO2) -> Sum1/1
  Art PO2/1 -> HB Bindung/1(PO2)
  Sum/1 -> Integrator/1
  Product/1 -> Sum/2

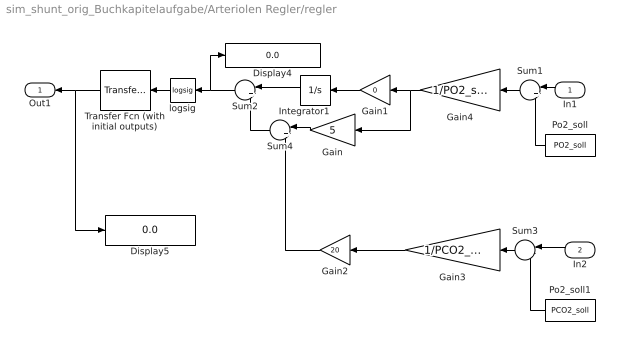
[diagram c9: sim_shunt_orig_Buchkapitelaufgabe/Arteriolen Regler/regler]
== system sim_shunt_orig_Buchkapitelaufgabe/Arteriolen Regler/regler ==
  In1 : Inport
  In2 : Inport  Port=2
  Display4 : Display
  Display5 : Display
  Gain : Gain  Gain=5
  Gain1 : Gain  Gain=0
  Gain2 : Gain  Gain=20
  Gain3 : Gain  Gain=1/PCO2_soll
  Gain4 : Gain  Gain=1/PO2_soll
  Integrator1 : Integrator  InitialCondition=ini2_reg  LimitOutput=on  UpperSaturationLimit=ini2_reg+0.2  LowerSaturationLimit=ini2_reg-0.2
  Po2_soll : Constant  Value=PO2_soll
  Po2_soll1 : Constant  Value=PCO2_soll
  Sum1 : Sum  Inputs=|+-
  Sum2 : Sum  Inputs=|++
  Sum3 : Sum  Inputs=|-+
  Sum4 : Sum  Inputs=|++
  Transfer Fcn (with initial outputs) : simulink_extras/Additional Linear/Transfer Fcn (with initial outputs)  N=[1]  D=[0.01 1]  Y0=A2_100  U0=A2_100
  logsig : neural/Transfer Functions/logsig
  Out1 : Outport
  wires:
  logsig/1 -> Transfer Fcn (with initial outputs)/1
  Integrator1/1 -> Sum2/1
  Gain1/1 -> Integrator1/1
  Gain/1 -> Sum4/1
  Gain2/1 -> Sum4/2
  Sum2/1 -> logsig/1, Display4/1
  Sum4/1 -> Sum2/2
  Transfer Fcn (with initial outputs)/1 -> Out1/1, Display5/1
  Po2_soll/1 -> Sum1/2
  In1/1 -> Sum1/1
  Sum1/1 -> Gain4/1
  Gain4/1 -> Gain/1, Gain1/1
  In2/1 -> Sum3/1
  Po2_soll1/1 -> Sum3/2
  Gain3/1 -> Gain2/1
  Sum3/1 -> Gain3/1

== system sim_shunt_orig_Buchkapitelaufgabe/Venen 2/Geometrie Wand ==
  r : Inport
  " " : Math  Operator=square
  "  " : Product  Inputs=***
  2 Korrekturfaktor : Gain
  Faktor : Constant  Value=2
  Summe : Sum  Inputs=+++
  Wurzel : Math  Operator=sqrt
  cm --> m : Gain  Gain=0.01
  "cm -> m" : Gain  Gain=0.01
  "h_1 " : Sum  Inputs=+-
  ho_1 : Constant  Value=h_0_ven
  r ^ 2 : Math  Operator=square
  ro_1 : Constant  Value=r_0_ven
  h : Outport
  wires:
  "h_1 "/1 -> h/1
  "  "/1 -> Summe/1
  Faktor/1 -> "  "/1
  ro_1/1 -> 2 Korrekturfaktor/1
  ho_1/1 -> cm --> m/1
  " "/1 -> Summe/2
  r ^ 2/1 -> Summe/3
  Wurzel/1 -> "h_1 "/1
  Summe/1 -> Wurzel/1
  r/1 -> r ^ 2/1, "h_1 "/2
  "cm -> m"/1 -> "  "/2
  cm --> m/1 -> "  "/3, " "/1
  2 Korrekturfaktor/1 -> "cm -> m"/1

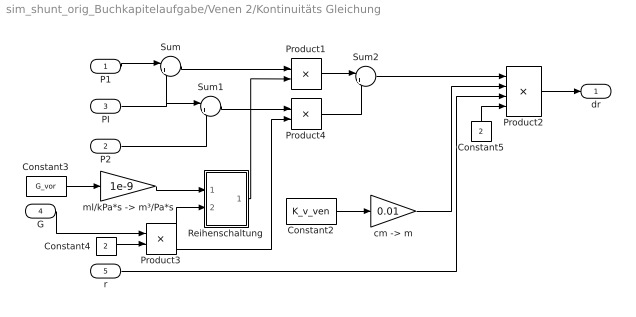
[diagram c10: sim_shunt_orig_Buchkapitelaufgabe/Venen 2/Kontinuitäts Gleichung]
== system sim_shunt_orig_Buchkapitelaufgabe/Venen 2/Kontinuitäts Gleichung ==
  P1 : Inport
  P2 : Inport  Port=2
  PI : Inport  Port=3
  G : Inport  Port=4
  r : Inport  Port=5
  Constant2 : Constant  Value=K_v_ven
  Constant3 : Constant  Value=G_vor
  Constant4 : Constant  Value=2
  Constant5 : Constant  Value=2
  Product1 : Product
  Product2 : Product  Inputs=*///
  Product3 : Product
  Product4 : Product
  Reihenschaltung : Subsystem
  Sum : Sum  Inputs=|+-
  Sum1 : Sum  Inputs=|+-
  Sum2 : Sum  Inputs=|+-
  "cm -> m" : Gain  Gain=0.01
  "ml/kPa*s -> m³/Pa*s" : Gain  Gain=1e-9
  dr : Outport
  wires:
  Constant5/1 -> Product2/4
  r/1 -> Product2/3
  Sum2/1 -> Product2/1
  Product4/1 -> Sum2/2
  Product3/1 -> Product4/2, Reihenschaltung/2(G2)
  Sum1/1 -> Product4/1
  Product1/1 -> Sum2/1
  Sum/1 -> Product1/1
  Constant2/1 -> "cm -> m"/1
  Product2/1 -> dr/1
  G/1 -> Product3/1
  Constant4/1 -> Product3/2
  Reihenschaltung/1(G_ges) -> Product1/2
  Constant3/1 -> "ml/kPa*s -> m³/Pa*s"/1
  PI/1 -> Sum1/1, Sum/2
  P2/1 -> Sum1/2
  P1/1 -> Sum/1
  "cm -> m"/1 -> Product2/2
  "ml/kPa*s -> m³/Pa*s"/1 -> Reihenschaltung/1(G1)

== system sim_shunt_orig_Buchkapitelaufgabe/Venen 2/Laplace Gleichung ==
  ICP : Inport
  Sigma : Inport  Port=2
  r : Inport  Port=3
  h : Inport  Port=4
  " " : Product  Inputs=**
  "  P_1" : Product  Inputs=*/
  " 1" : Product  Inputs=**
  Summe : Sum
  r +h : Sum
  PI : Outport
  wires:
  "  P_1"/1 -> PI/1
  h/1 -> " 1"/2, r +h/2
  Sigma/1 -> " 1"/1
  r/1 -> r +h/1, "  P_1"/2
  ICP/1 -> " "/1
  r +h/1 -> " "/2
  " 1"/1 -> Summe/1
  Summe/1 -> "  P_1"/1
  " "/1 -> Summe/2

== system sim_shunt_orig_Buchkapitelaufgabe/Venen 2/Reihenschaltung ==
  G1 : Inport
  G2 : Inport  Port=2
  Fcn : Fcn  Expr=(u(1)*u(2))/(u(1)+u(2))
  Mux : Mux  Inputs=2
  G_ges : Outport
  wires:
  G1/1 -> Mux/1
  G2/1 -> Mux/2
  Mux/1 -> Fcn/1
  Fcn/1 -> G_ges/1

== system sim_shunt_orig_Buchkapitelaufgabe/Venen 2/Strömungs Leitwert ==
  r : Inport
  1/kPa*cm*s v 1/Pa*s*m : Gain  Gain=0.1
  Leitwert Konstante : Constant  Value=K_G_ven
  Potenz : Constant  Value=4
  Product : Product
  r ^ 4 : Math  Operator=pow
  G : Outport
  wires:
  Product/1 -> G/1
  r/1 -> r ^ 4/1
  Leitwert Konstante/1 -> 1/kPa*cm*s v 1/Pa*s*m/1
  r ^ 4/1 -> Product/1
  Potenz/1 -> r ^ 4/2
  1/kPa*cm*s v 1/Pa*s*m/1 -> Product/2

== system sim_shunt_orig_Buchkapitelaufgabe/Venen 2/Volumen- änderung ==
  dr : Inport
  r : Inport  Port=2
  Faktor : Constant  Value=2
  Kv_1 : Constant  Value=K_v_ven
  "cm -> m" : Gain  Gain=0.01
  "dV_1 " : Product  Inputs=4
  dV : Outport
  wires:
  "dV_1 "/1 -> dV/1
  Faktor/1 -> "dV_1 "/1
  Kv_1/1 -> "cm -> m"/1
  dr/1 -> "dV_1 "/3
  r/1 -> "dV_1 "/4
  "cm -> m"/1 -> "dV_1 "/2

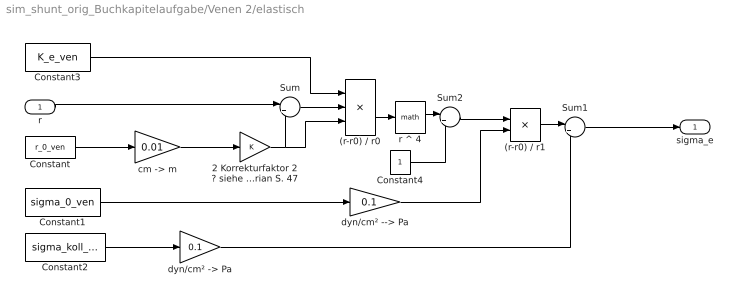
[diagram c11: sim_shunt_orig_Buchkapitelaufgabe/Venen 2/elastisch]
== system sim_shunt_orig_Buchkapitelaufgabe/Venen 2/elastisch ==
  r : Inport
  (r-r0) / r0 : Product  Inputs=**/
  (r-r0) / r1 : Product
  2 Korrekturfaktor 2 ? siehe Diss. Marian S. 47 : Gain
  Constant : Constant  Value=r_0_ven
  Constant1 : Constant  Value=sigma_0_ven
  Constant2 : Constant  Value=sigma_koll_ven
  Constant3 : Constant  Value=K_e_ven
  Constant4 : Constant
  Sum : Sum  Inputs=|+-
  Sum1 : Sum  Inputs=|+-
  Sum2 : Sum  Inputs=|+-
  "cm -> m" : Gain  Gain=0.01
  dyn/cm² --> Pa : Gain  Gain=0.1
  "dyn/cm² -> Pa" : Gain  Gain=0.1
  r ^ 4 : Math
  sigma_e : Outport
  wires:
  (r-r0) / r0/1 -> r ^ 4/1
  Sum/1 -> (r-r0) / r0/2
  Constant3/1 -> (r-r0) / r0/1
  (r-r0) / r1/1 -> Sum1/1
  r/1 -> Sum/1
  Sum1/1 -> sigma_e/1
  Constant2/1 -> "dyn/cm² -> Pa"/1
  Constant1/1 -> dyn/cm² --> Pa/1
  r ^ 4/1 -> Sum2/1
  Sum2/1 -> (r-r0) / r1/1
  Constant4/1 -> Sum2/2
  "cm -> m"/1 -> 2 Korrekturfaktor 2 ? siehe Diss. Marian S. 47/1
  "dyn/cm² -> Pa"/1 -> Sum1/2
  dyn/cm² --> Pa/1 -> (r-r0) / r1/2
  2 Korrekturfaktor 2 ? siehe Diss. Marian S. 47/1 -> (r-r0) / r0/3, Sum/2
  Constant/1 -> "cm -> m"/1

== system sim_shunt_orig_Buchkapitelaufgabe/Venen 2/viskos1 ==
  dr : Inport
  Constant2 : Constant  Value=sigma_0_visk_2
  Product : Product
  Transfer Fcn : TransferFcn  Denominator=[0.01 1]
  dyn*s/cm³ v Pa*s/m : Gain  Gain=10
  sigma_v : Outport
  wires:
  Product/1 -> sigma_v/1
  dr/1 -> Transfer Fcn/1
  Constant2/1 -> dyn*s/cm³ v Pa*s/m/1
  Transfer Fcn/1 -> Product/1
  dyn*s/cm³ v Pa*s/m/1 -> Product/2

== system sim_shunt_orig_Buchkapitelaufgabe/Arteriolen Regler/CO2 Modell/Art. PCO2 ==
  Art PCO2 : Constant  Value=41
  Art PO4 : Constant  Value=0
  Art PO5 : Constant  Value=0.04
  Clock : Clock
  Manual Switch : ManualSwitch
  Product2 : Product
  Scope : Scope
  Signal Generator : SignalGenerator  WaveForm=sawtooth  Amplitude=0.04  Frequency=0.005
  Sum3 : Sum  Inputs=|++
  Sum4 : Sum  Inputs=|+-
  Switch1 : Switch  Threshold=400
  Out1 : Outport
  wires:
  Art PCO2/1 -> Sum3/1, Product2/1, Scope/1
  Sum4/1 -> Product2/2
  Signal Generator/1 -> Sum4/2
  Art PO5/1 -> Sum4/1
  Clock/1 -> Switch1/2
  Product2/1 -> Switch1/1
  Art PO4/1 -> Switch1/3, Manual Switch/2
  Switch1/1 -> Manual Switch/1
  Manual Switch/1 -> Sum3/2
  Sum3/1 -> Out1/1

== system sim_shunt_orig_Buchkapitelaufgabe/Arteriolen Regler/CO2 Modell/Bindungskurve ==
  PCO2 : Inport
  PO2 : Inport  Port=2
  CBF : Constant  Value=1.2095
  CBF1 : Constant  Value=100
  Display1 : Display
  Display2 : Display
  OG : Subsystem
  Product : Product  Inputs=*/
  Product1 : Product
  Sum1 : Sum  Inputs=|+-
  Sum2 : Sum  Inputs=|++
  Sum3 : Sum  Inputs=|+-
  UG : Subsystem
  MCO2 : Outport
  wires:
  UG/1(MCO2) -> Display2/1, Sum2/2, Sum1/2
  OG/1(MCO2) -> Display1/1, Sum1/1
  Sum2/1 -> MCO2/1
  Product1/1 -> Sum2/1
  Sum1/1 -> Product1/2
  Sum3/1 -> Product1/1
  Product/1 -> Sum3/2
  CBF/1 -> Sum3/1
  CBF1/1 -> Product/2
  PO2/1 -> Product/1
  PCO2/1 -> UG/1(PCO2), OG/1(PCO2)

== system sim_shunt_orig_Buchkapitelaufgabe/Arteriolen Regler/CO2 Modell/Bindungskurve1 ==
  PCO2 : Inport
  PO2 : Inport  Port=2
  CBF : Constant  Value=1.4
  CBF1 : Constant  Value=100
  Display{3..7} (5 alike) : Display
  OG : Subsystem
  Product : Product  Inputs=*/
  Product1 : Product
  Sum1 : Sum  Inputs=|+-
  Sum2 : Sum  Inputs=|++
  Sum3 : Sum  Inputs=|+-
  UG : Subsystem
  MCO2 : Outport
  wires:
  Sum2/1 -> Display7/1, MCO2/1
  Product1/1 -> Display6/1, Sum2/1
  Sum3/1 -> Display5/1, Product1/1
  OG/1(MCO2) -> Display4/1, Sum1/1
  UG/1(MCO2) -> Display3/1, Sum1/2, Sum2/2
  PCO2/1 -> OG/1(PCO2), UG/1(PCO2)
  PO2/1 -> Product/1
  CBF1/1 -> Product/2
  CBF/1 -> Sum3/1
  Product/1 -> Sum3/2
  Sum1/1 -> Product1/2

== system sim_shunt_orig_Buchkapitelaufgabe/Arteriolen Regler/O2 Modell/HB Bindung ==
  PO2 : Inport  PortDimensions=1
  Layer 1 : Subsystem
  Layer 2 : Subsystem
  MO2 : Outport  InitialOutput=0
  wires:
  PO2/1 -> Layer 1/1("p{1}")
  Layer 1/1("a{1}") -> [feedback1]
  [feedback1] -> Layer 2/1("a{1} ")
  Layer 2/1("a{2}") -> MO2/1

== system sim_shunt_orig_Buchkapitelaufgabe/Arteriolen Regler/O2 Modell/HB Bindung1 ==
  PO2 : Inport  PortDimensions=1
  Layer 1 : Subsystem
  Layer 2 : Subsystem
  MO2 : Outport  InitialOutput=0
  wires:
  Layer 2/1("a{2}") -> MO2/1
  [feedback1] -> Layer 2/1("a{1} ")
  Layer 1/1("a{1}") -> [feedback1]
  PO2/1 -> Layer 1/1("p{1}")

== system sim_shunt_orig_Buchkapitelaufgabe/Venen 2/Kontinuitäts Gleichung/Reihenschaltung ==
  G1 : Inport
  G2 : Inport  Port=2
  Fcn : Fcn  Expr=(u(1)*u(2))/(u(1)+u(2))
  Mux : Mux  Inputs=2
  G_ges : Outport
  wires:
  Fcn/1 -> G_ges/1
  Mux/1 -> Fcn/1
  G2/1 -> Mux/2
  G1/1 -> Mux/1

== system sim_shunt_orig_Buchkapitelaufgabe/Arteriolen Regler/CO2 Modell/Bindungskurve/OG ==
  PCO2 : Inport  PortDimensions=1
  Layer 1 : Subsystem
  Layer 2 : Subsystem
  MCO2 : Outport  InitialOutput=0
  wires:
  Layer 2/1("a{2}") -> MCO2/1
  [feedback1] -> Layer 2/1("a{1} ")
  Layer 1/1("a{1}") -> [feedback1]
  PCO2/1 -> Layer 1/1("p{1}")

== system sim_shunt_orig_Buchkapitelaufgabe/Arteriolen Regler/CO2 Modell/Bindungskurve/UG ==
  PCO2 : Inport  PortDimensions=1
  Layer 1 : Subsystem
  Layer 2 : Subsystem
  Saturation : Saturate  UpperLimit=2000  LowerLimit=0
  MCO2 : Outport  InitialOutput=0
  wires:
  Saturation/1 -> MCO2/1
  Layer 2/1("a{2}") -> Saturation/1
  [feedback1] -> Layer 2/1("a{1} ")
  Layer 1/1("a{1}") -> [feedback1]
  PCO2/1 -> Layer 1/1("p{1}")

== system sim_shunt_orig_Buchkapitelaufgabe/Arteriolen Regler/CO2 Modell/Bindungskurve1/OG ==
  PCO2 : Inport  PortDimensions=1
  Layer 1 : Subsystem
  Layer 2 : Subsystem
  MCO2 : Outport  InitialOutput=0
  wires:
  PCO2/1 -> Layer 1/1("p{1}")
  Layer 1/1("a{1}") -> [feedback1]
  [feedback1] -> Layer 2/1("a{1} ")
  Layer 2/1("a{2}") -> MCO2/1

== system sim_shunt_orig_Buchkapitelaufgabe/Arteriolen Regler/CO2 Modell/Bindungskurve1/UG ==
  PCO2 : Inport  PortDimensions=1
  Layer 1 : Subsystem
  Layer 2 : Subsystem
  Saturation : Saturate  UpperLimit=2000  LowerLimit=0
  MCO2 : Outport  InitialOutput=0
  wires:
  PCO2/1 -> Layer 1/1("p{1}")
  Layer 1/1("a{1}") -> [feedback1]
  [feedback1] -> Layer 2/1("a{1} ")
  Layer 2/1("a{2}") -> Saturation/1
  Saturation/1 -> MCO2/1

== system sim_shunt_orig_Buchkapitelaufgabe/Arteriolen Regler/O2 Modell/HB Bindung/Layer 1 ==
  "p{1}" : Inport  PortDimensions=1
  Delays 1 : Subsystem
  "IW{1,1}" : Subsystem
  "b{1}" : Constant  Value=[0.56940775501339358;0.74992370778593587]
  logsig : neural/Transfer Functions/logsig
  netsum : Sum  Inputs=2
  "a{1}" : Outport  InitialOutput=[0;0]
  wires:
  "p{1}"/1 -> Delays 1/1("p{1}")
  Delays 1/1("pd{1,1}") -> "IW{1,1}"/1("pd{1,1}")
  "IW{1,1}"/1("iz{1,1}") -> netsum/1
  "b{1}"/1 -> netsum/2
  netsum/1 -> logsig/1
  logsig/1 -> "a{1}"/1

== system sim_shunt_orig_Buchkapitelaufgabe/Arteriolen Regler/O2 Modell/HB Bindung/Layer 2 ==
  "a{1} " : Inport  PortDimensions=2
  Delays 1 : Subsystem
  "LW{2,1}" : Subsystem
  "b{2}" : Constant  Value=9.3385368948146255
  netsum : Sum  Inputs=2
  purelin : neural/Transfer Functions/purelin
  "a{2}" : Outport  InitialOutput=0
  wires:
  "a{1} "/1 -> Delays 1/1("p{2}")
  Delays 1/1("pd{2,1}") -> "LW{2,1}"/1("ad{2,1}")
  "LW{2,1}"/1("lz{2,1}") -> netsum/1
  "b{2}"/1 -> netsum/2
  netsum/1 -> purelin/1
  purelin/1 -> "a{2}"/1

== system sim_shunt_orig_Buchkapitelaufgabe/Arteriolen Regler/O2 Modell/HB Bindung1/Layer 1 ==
  "p{1}" : Inport  PortDimensions=1
  Delays 1 : Subsystem
  "IW{1,1}" : Subsystem
  "b{1}" : Constant  Value=[0.56940775501339358;0.74992370778593587]
  logsig : neural/Transfer Functions/logsig
  netsum : Sum  Inputs=2
  "a{1}" : Outport  InitialOutput=[0;0]
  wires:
  logsig/1 -> "a{1}"/1
  netsum/1 -> logsig/1
  "b{1}"/1 -> netsum/2
  "IW{1,1}"/1("iz{1,1}") -> netsum/1
  Delays 1/1("pd{1,1}") -> "IW{1,1}"/1("pd{1,1}")
  "p{1}"/1 -> Delays 1/1("p{1}")

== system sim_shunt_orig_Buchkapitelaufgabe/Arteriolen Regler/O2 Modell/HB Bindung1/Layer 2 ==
  "a{1} " : Inport  PortDimensions=2
  Delays 1 : Subsystem
  "LW{2,1}" : Subsystem
  "b{2}" : Constant  Value=9.3385368948146255
  netsum : Sum  Inputs=2
  purelin : neural/Transfer Functions/purelin
  "a{2}" : Outport  InitialOutput=0
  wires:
  purelin/1 -> "a{2}"/1
  netsum/1 -> purelin/1
  "b{2}"/1 -> netsum/2
  "LW{2,1}"/1("lz{2,1}") -> netsum/1
  Delays 1/1("pd{2,1}") -> "LW{2,1}"/1("ad{2,1}")
  "a{1} "/1 -> Delays 1/1("p{2}")

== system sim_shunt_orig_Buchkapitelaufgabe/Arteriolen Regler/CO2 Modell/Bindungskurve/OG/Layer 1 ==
  "p{1}" : Inport  PortDimensions=1
  Delays 1 : Subsystem
  "IW{1,1}" : Subsystem
  "b{1}" : Constant  Value=[21.466440059106699;0.55998995039437871;1.7651126643638742]
  logsig : neural/Transfer Functions/logsig
  netsum : Sum  Inputs=2
  "a{1}" : Outport  InitialOutput=[0;0;0]
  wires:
  logsig/1 -> "a{1}"/1
  netsum/1 -> logsig/1
  "b{1}"/1 -> netsum/2
  "IW{1,1}"/1("iz{1,1}") -> netsum/1
  Delays 1/1("pd{1,1}") -> "IW{1,1}"/1("pd{1,1}")
  "p{1}"/1 -> Delays 1/1("p{1}")

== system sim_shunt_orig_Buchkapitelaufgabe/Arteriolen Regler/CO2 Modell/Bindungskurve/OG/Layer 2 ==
  "a{1} " : Inport  PortDimensions=3
  Delays 1 : Subsystem
  "LW{2,1}" : Subsystem
  "b{2}" : Constant  Value=-57.1363139852579
  netsum : Sum  Inputs=2
  purelin : neural/Transfer Functions/purelin
  "a{2}" : Outport  InitialOutput=0
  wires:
  purelin/1 -> "a{2}"/1
  netsum/1 -> purelin/1
  "b{2}"/1 -> netsum/2
  "LW{2,1}"/1("lz{2,1}") -> netsum/1
  Delays 1/1("pd{2,1}") -> "LW{2,1}"/1("ad{2,1}")
  "a{1} "/1 -> Delays 1/1("p{2}")

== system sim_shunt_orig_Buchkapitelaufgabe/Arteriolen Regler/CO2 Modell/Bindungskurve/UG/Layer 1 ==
  "p{1}" : Inport  PortDimensions=1
  Delays 1 : Subsystem
  "IW{1,1}" : Subsystem
  "b{1}" : Constant  Value=[-0.93928791775244591;-3.2355235792872823;-1.3419689885961057]
  logsig : neural/Transfer Functions/logsig
  netsum : Sum  Inputs=2
  "a{1}" : Outport  InitialOutput=[0;0;0]
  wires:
  logsig/1 -> "a{1}"/1
  netsum/1 -> logsig/1
  "b{1}"/1 -> netsum/2
  "IW{1,1}"/1("iz{1,1}") -> netsum/1
  Delays 1/1("pd{1,1}") -> "IW{1,1}"/1("pd{1,1}")
  "p{1}"/1 -> Delays 1/1("p{1}")

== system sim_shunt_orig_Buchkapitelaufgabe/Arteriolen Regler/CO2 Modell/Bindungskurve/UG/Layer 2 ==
  "a{1} " : Inport  PortDimensions=3
  Delays 1 : Subsystem
  "LW{2,1}" : Subsystem
  "b{2}" : Constant  Value=-10.767514147651568
  netsum : Sum  Inputs=2
  purelin : neural/Transfer Functions/purelin
  "a{2}" : Outport  InitialOutput=0
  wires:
  purelin/1 -> "a{2}"/1
  netsum/1 -> purelin/1
  "b{2}"/1 -> netsum/2
  "LW{2,1}"/1("lz{2,1}") -> netsum/1
  Delays 1/1("pd{2,1}") -> "LW{2,1}"/1("ad{2,1}")
  "a{1} "/1 -> Delays 1/1("p{2}")

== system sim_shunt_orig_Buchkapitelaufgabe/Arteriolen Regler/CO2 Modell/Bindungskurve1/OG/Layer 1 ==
  "p{1}" : Inport  PortDimensions=1
  Delays 1 : Subsystem
  "IW{1,1}" : Subsystem
  "b{1}" : Constant  Value=[21.466440059106699;0.55998995039437871;1.7651126643638742]
  logsig : neural/Transfer Functions/logsig
  netsum : Sum  Inputs=2
  "a{1}" : Outport  InitialOutput=[0;0;0]
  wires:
  "p{1}"/1 -> Delays 1/1("p{1}")
  Delays 1/1("pd{1,1}") -> "IW{1,1}"/1("pd{1,1}")
  "IW{1,1}"/1("iz{1,1}") -> netsum/1
  "b{1}"/1 -> netsum/2
  netsum/1 -> logsig/1
  logsig/1 -> "a{1}"/1

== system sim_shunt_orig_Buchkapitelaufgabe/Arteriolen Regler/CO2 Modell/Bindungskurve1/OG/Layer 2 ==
  "a{1} " : Inport  PortDimensions=3
  Delays 1 : Subsystem
  "LW{2,1}" : Subsystem
  "b{2}" : Constant  Value=-57.1363139852579
  netsum : Sum  Inputs=2
  purelin : neural/Transfer Functions/purelin
  "a{2}" : Outport  InitialOutput=0
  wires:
  "a{1} "/1 -> Delays 1/1("p{2}")
  Delays 1/1("pd{2,1}") -> "LW{2,1}"/1("ad{2,1}")
  "LW{2,1}"/1("lz{2,1}") -> netsum/1
  "b{2}"/1 -> netsum/2
  netsum/1 -> purelin/1
  purelin/1 -> "a{2}"/1

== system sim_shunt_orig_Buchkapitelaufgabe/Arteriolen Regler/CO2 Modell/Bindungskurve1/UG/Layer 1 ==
  "p{1}" : Inport  PortDimensions=1
  Delays 1 : Subsystem
  "IW{1,1}" : Subsystem
  "b{1}" : Constant  Value=[-0.93928791775244591;-3.2355235792872823;-1.3419689885961057]
  logsig : neural/Transfer Functions/logsig
  netsum : Sum  Inputs=2
  "a{1}" : Outport  InitialOutput=[0;0;0]
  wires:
  "p{1}"/1 -> Delays 1/1("p{1}")
  Delays 1/1("pd{1,1}") -> "IW{1,1}"/1("pd{1,1}")
  "IW{1,1}"/1("iz{1,1}") -> netsum/1
  "b{1}"/1 -> netsum/2
  netsum/1 -> logsig/1
  logsig/1 -> "a{1}"/1

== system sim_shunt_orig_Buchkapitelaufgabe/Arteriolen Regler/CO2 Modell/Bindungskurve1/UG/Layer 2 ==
  "a{1} " : Inport  PortDimensions=3
  Delays 1 : Subsystem
  "LW{2,1}" : Subsystem
  "b{2}" : Constant  Value=-10.767514147651568
  netsum : Sum  Inputs=2
  purelin : neural/Transfer Functions/purelin
  "a{2}" : Outport  InitialOutput=0
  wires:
  "a{1} "/1 -> Delays 1/1("p{2}")
  Delays 1/1("pd{2,1}") -> "LW{2,1}"/1("ad{2,1}")
  "LW{2,1}"/1("lz{2,1}") -> netsum/1
  "b{2}"/1 -> netsum/2
  netsum/1 -> purelin/1
  purelin/1 -> "a{2}"/1
